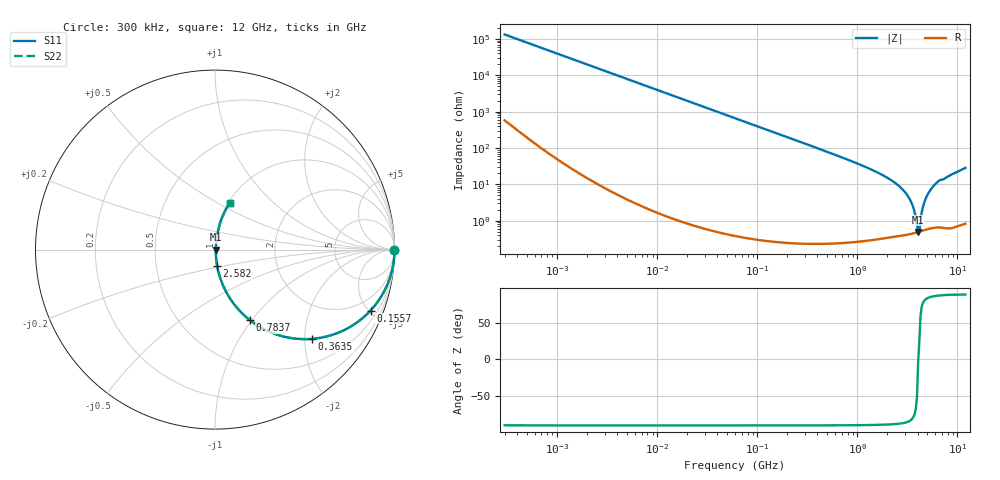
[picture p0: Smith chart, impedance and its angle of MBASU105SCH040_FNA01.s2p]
! MBASU105SCH040_FNA01  S-PARAMETER MODEL  ( Standard Model )
! Model Generated by TAIYO YUDEN Corporation (http://www.ty-top.com)
! Version 1.0
! TAIYO YUDEN Control No. 230609
! Copyright(c) 2023 TAIYO YUDEN CO.,LTD. All Rights Reserved.
! Product Description (link to TY-COMPAS)
! https://ds.yuden.co.jp/TYCOMPAS/or/detail?pn=MBASU105SCH040BFNA01&u=M
! Products Name : Multilayer Ceramic Capacitors
! Characteristics :
!  Capacitance : 4 [pF] , Rated Voltage : 50 [V] , TCC : CH / C0H
!  Case Size : 1.0 x 0.5 / 0.039 x 0.02 [mm/inch] , Thickness : 0.5 / 0.02 [mm/inch]
!  (Conditions: Temperature = 25 [degC] , DC Bias Voltage = 0 [V])
! External Node Assignments :
!  1  o---| |---o  2
! GND o---------o GND
! Frequency Range : 0.3MHz  -  12000MHz  [ 401 STEP ]
# MHZ S RI R 50
! Freq[MHz].  S11 Real  S11 Imag  S21 Real  S21 Imag  S12 Real  S12 Imag  S22 Real  S22 Imag
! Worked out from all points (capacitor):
!   401 points, 300 kHz to 12 GHz, reference 50 ohm
!   read as one part in series: C = 4 pF near 316.3 kHz
!   lowest |Z| = 489 mohm at 4.05 GHz (marker M1)
!   series resonance near 4.062 GHz, so ESL is about 380 pH
!   S11 on the Smith chart (normalised r, x): 300 kHz: open; 155.7 MHz: 1.01, -5.10; 363.5 MHz: 1.00, -2.17; 783.7 MHz: 1.00, -0.98; 2.582 GHz: 1.01, -0.18; 12 GHz: 1.02, +0.57
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0.3  1 -0.000754  3.83e-06 0.000754  3.83e-06 0.000754  1 -0.000754
1.769972  1 -0.00445  2.34e-05 0.00445  2.34e-05 0.00445  1 -0.00445
10.44266  0.9993 -0.0262  0.000699 0.0262  0.000699 0.0262  0.9993 -0.0262
60  0.9777 -0.1474  0.0223 0.1474  0.0223 0.1474  0.9777 -0.1474
155.7172  0.8666 -0.3395  0.1334 0.3395  0.1334 0.3395  0.8666 -0.3395
353.9943  0.5543 -0.496  0.4457 0.496  0.4457 0.496  0.5543 -0.496
363.4975  0.541 -0.4973  0.459 0.4973  0.459 0.4973  0.541 -0.4973
783.7017  0.1941 -0.393  0.8059 0.393  0.8059 0.393  0.1941 -0.393
2088.533  0.0225 -0.1366  0.9775 0.1366  0.9775 0.1366  0.0225 -0.1366
2581.562  0.012 -0.0905  0.988 0.0905  0.988 0.0905  0.012 -0.0905
3026.31  0.00737 -0.0579  0.9926 0.0579  0.9926 0.0579  0.00737 -0.0579
3364.605  0.00561 -0.0368  0.9944 0.0368  0.9944 0.0368  0.00561 -0.0368
3642.919  0.00493 -0.0212  0.9951 0.0212  0.9951 0.0212  0.00493 -0.0212
3944.255  0.00479 -0.00576  0.9952 0.00576  0.9952 0.00576  0.00479 -0.00576
4050.141  0.00486 -0.00027  0.9951 0.00027  0.9951 0.00027  0.00486 -0.00027
4270.516  0.00514 0.00817  0.9949 -0.00817  0.9949 -0.00817  0.00514 0.00817
4502.883  0.00579 0.0218  0.9942 -0.0218  0.9942 -0.0218  0.00579 0.0218
4747.894  0.00683 0.0356  0.9932 -0.0356  0.9932 -0.0356  0.00683 0.0356
5140.631  0.00916 0.0568  0.9908 -0.0568  0.9908 -0.0568  0.00916 0.0568
5715.274  0.0137 0.0855  0.9863 -0.0855  0.9863 -0.0855  0.0137 0.0855
6699.894  0.0229 0.1267  0.9771 -0.1267  0.9771 -0.1267  0.0229 0.1267
12000  0.0813 0.2591  0.9187 -0.2591  0.9187 -0.2591  0.0813 0.2591
